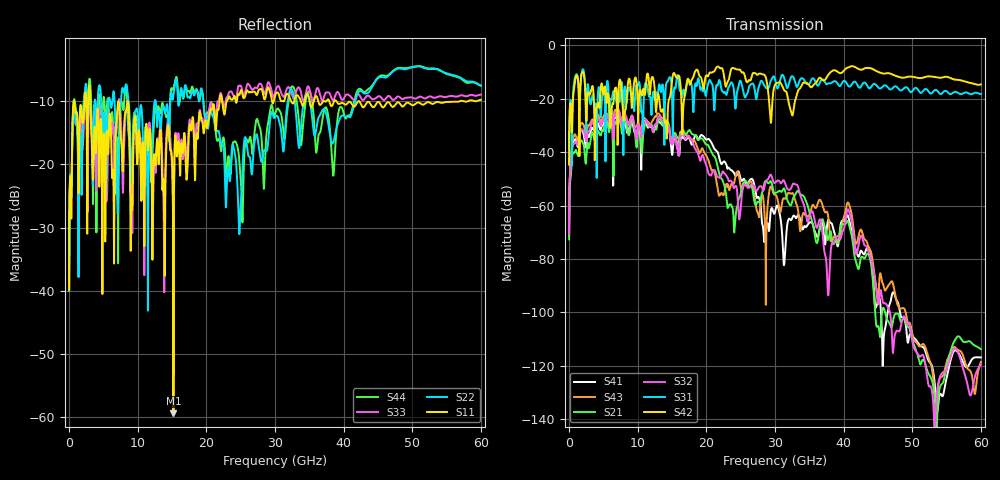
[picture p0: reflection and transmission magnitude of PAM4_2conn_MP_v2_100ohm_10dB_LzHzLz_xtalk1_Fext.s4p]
! Info: Touchstone file created by Circ.  Input file=FAB50GbE_2conn_Midplane_Examax_Topo2_v2_100ohm_10dB_LzHzLz.circ
# Hz S RI R 50
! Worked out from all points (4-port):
!   6000 points, 10 MHz to 60 GHz, reference 50 ohm
!   strongest paths, dB at 10 MHz, 15.01 GHz, 30.01 GHz, 45.01 GHz, 60 GHz:
!     S42: -44.7, -13.0, -14.7, -9.9, -14.7
!     S31: -44.0, -19.6, -12.6, -15.7, -18.2
!     S32: -70.7, -37.1, -51.5, -95.6, -119.5
!     S21: -72.7, -36.4, -55.4, -105.1, -113.8
!     S43: -71.4, -36.3, -56.0, -95.9, -118.5
!     S41: -67.7, -41.0, -62.4, -95.7, -116.9
!   lowest |S11| = -59.4 dB at 15.21 GHz (marker M1), VSWR 1.00, Z = 49.9 + j0.0857 ohm
!   |S11| at or under -10 dB: 3.12 GHz to 7.187 GHz (4.067 GHz wide, 78.9 % of centre); 8.589 GHz to 21.92 GHz (13.34 GHz wide, 87.4 % of centre); 42.29 GHz to 56.86 GHz (14.57 GHz wide, 29.4 % of centre)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
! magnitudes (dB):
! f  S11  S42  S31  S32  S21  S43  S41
! 10 MHz  -39.8  -44.7  -44.0  -70.7  -72.7  -71.4  -67.7
! 1.86 GHz  -12.5  -10.4  -10.0  -31.5  -35.7  -29.0  -31.6
! 15.21 GHz  -59.4  -10.5  -20.2  -35.0  -35.2  -33.1  -36.3
! 24.09 GHz  -9.2  -8.6  -18.9  -53.2  -69.6  -51.2  -48.0
! 31.34 GHz  -9.9  -16.8  -12.2  -50.7  -53.7  -57.2  -82.1
! 37.71 GHz  -9.7  -11.3  -14.3  -92.5  -72.9  -63.3  -65.7
! 60 GHz  -9.8  -14.7  -18.2  -119.5  -113.8  -118.5  -116.9
